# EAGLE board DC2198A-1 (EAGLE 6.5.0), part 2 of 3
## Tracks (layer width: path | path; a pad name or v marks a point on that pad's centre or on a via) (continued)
GND  (via drill 0.25) (continued)
  pour Top (no thermals): 50.29,32 46.74,32 46.74,35.31 51.56,35.31 52.2,34.67 52.2,33.02 51.56,33.02 51.56,34.42 51.31,34.67 50.55,34.67 50.29,34.42
  pour Bottom (no thermals): 50.29,32 46.74,32 46.74,35.18 49.91,35.18 50.29,34.8
  pour Bottom (no thermals): 69.6,41.27 69.6,36.58 67.44,36.58 67.06,36.2 67.06,35.05 65.15,35.05 65.15,36.58 65.53,36.96 65.53,40.26 66.55,41.27
  pour Top (no thermals): 61.85,32 58.29,32 58.29,35.31 63.12,35.31 63.75,34.67 63.75,33.02 63.12,33.02 63.12,34.42 62.87,34.67 62.1,34.67 61.85,34.42
  pour Bottom (no thermals): 61.85,32 58.29,32 58.29,35.18 61.47,35.18 61.85,34.8
  pour Bottom (no thermals): 81.15,41.27 81.15,36.58 78.99,36.58 78.61,36.2 78.61,35.05 76.71,35.05 76.71,36.58 77.09,36.96 77.09,40.26 78.11,41.27
  pour Top (no thermals): 73.41,32 69.85,32 69.85,35.31 74.68,35.31 75.31,34.67 75.31,33.02 74.68,33.02 74.68,34.42 74.42,34.67 73.66,34.67 73.41,34.42
  pour Bottom (no thermals): 73.41,32 69.85,32 69.85,35.18 73.03,35.18 73.41,34.8
  pour Bottom (no thermals): 92.71,41.27 92.71,36.58 90.55,36.58 90.17,36.2 90.17,35.05 88.27,35.05 88.27,36.58 88.65,36.96 88.65,40.26 89.66,41.27
  pour Top (no thermals): 84.96,32 81.41,32 81.41,35.31 86.23,35.31 86.87,34.67 86.87,33.02 86.23,33.02 86.23,34.42 85.98,34.67 85.22,34.67 84.96,34.42
  pour Bottom (no thermals): 84.96,32 81.41,32 81.41,35.18 84.58,35.18 84.96,34.8
  pour Bottom (no thermals): 104.27,41.27 104.27,36.58 102.11,36.58 101.73,36.2 101.73,35.05 99.82,35.05 99.82,36.58 100.2,36.96 100.2,40.26 101.22,41.27
  pour Top (no thermals): 96.52,32 92.96,32 92.96,35.31 97.79,35.31 98.42,34.67 98.42,33.02 97.79,33.02 97.79,34.42 97.54,34.67 96.77,34.67 96.52,34.42
  pour Bottom (no thermals): 96.52,32 92.96,32 92.96,35.18 96.14,35.18 96.52,34.8
  pour Top: 50.29,30.86 65.91,30.86 65.91,14.35 50.29,14.35
IBV_AUX  (via drill 0.25)
  Top 0.203: C20.1 110.4,24.42 110.57,24.59 112.47,24.59 113.03,25.15 113.03,26.04 112.14,26.92 112.14,27.34 U9.8 | 107.95,27.51 107.95,25.02 | U11.1 117.19,20.77 C25.1 | v113.41,21.21 113.41,21.03 114.17,20.77
  Top 0.254: U11.1 U11.2
  Top 0.406: C20.1 110.28,23.75 R28.2 108.71,22.23 108.08,22.23 108.08,22.99 C21.1 107.95,22.99 107.95,27.51 L9.2
  Top 1.016: 113.1,20.77 114.17,20.77 U11.1 | 108.71,22.23 108.71,21.59 109.78,20.77 113.1,20.77 | R30.2 113.2,20.73 113.16,20.83 113.1,20.77
  Bottom 0.406: D1.1 113.43,21.1 v113.41,21.21
  pour Top (no thermals): 107.06,19.81 107.06,26.42 106.68,26.8 105.66,26.8 105.66,28.32 107.82,28.32 108.33,27.81 108.33,24.51 111,24.51 111,21.46 119.38,21.46 119.38,19.94 119.25,19.81
INTVCC_LTC3604  (via drill 0.25)
  Top 0.203: v112.27,25.73 112.27,26.16 111.63,26.8 111.63,27.33 U9.7 | U9.1 108.99,29.94 108.97,29.97 v108.97,30.61 | U9.10 113.8,28.94 113.92,28.83 v113.92,25.4
  Bottom 0.203: C67.1 115.19,27.22 115.15,27.18 113.92,27.18 | 112.27,27.18 v112.27,25.73 | 112.27,27.18 109.09,27.18 108.97,27.3 v108.97,30.61 | 112.27,27.18 113.92,27.18 | 113.92,27.18 v113.92,25.4
ITH_LTC3604  (via drill 0.25)
  Top 0.203: U9.12 113.89,29.94 114.05,30.1 v114.05,30.86
  Bottom 0.203: v114.05,30.86 113.79,30.86 113.79,28.83 112.78,28.83 | 112.74,28.83 R102.2 112.78,28.83 | C68.1 110.49,28.57 112.78,28.57 112.78,28.83
N$1
  Top 0.406: P1.P 12.19,43.05 12.19,40.77 12.95,40.77 R17.1
N$2  (via drill 0.25)
  Top 0.203: v15.49,43.69 15.11,43.31 14.59,43.31 P1.N
  Bottom 0.203: v15.49,43.69 14.22,43.69 14.22,42.67 Q17.3
N$3
  Top 0.406: R26.2 LED1.P
N$4
  Top 0.406: P2.P 23.75,43.05 23.75,40.77 24.51,40.77 R18.1
N$5  (via drill 0.25)
  Top 0.203: v27.05,43.69 26.67,43.31 26.15,43.31 P2.N
  Bottom 0.203: v27.05,43.69 25.78,43.69 25.78,42.67 Q16.3
N$6
  Top 0.406: P3.P 35.31,43.05 35.31,40.77 36.07,40.77 R19.1
N$7  (via drill 0.25)
  Top 0.203: v38.61,43.69 38.23,43.31 37.71,43.31 P3.N
  Bottom 0.203: v38.61,43.69 37.34,43.69 37.34,42.67 Q15.3
N$8
  Top 0.406: P4.P 46.86,43.05 46.86,40.77 47.62,40.77 R20.1
N$9  (via drill 0.25)
  Top 0.203: v50.16,43.69 49.78,43.31 49.26,43.31 P4.N
  Bottom 0.203: v50.16,43.69 48.9,43.69 48.9,42.67 Q14.3
N$10
  Top 0.406: P5.P 58.42,43.05 58.42,40.77 59.18,40.77 R21.1
N$11  (via drill 0.25)
  Top 0.203: v61.72,43.69 61.34,43.31 60.82,43.31 P5.N
  Bottom 0.203: v61.72,43.69 60.45,43.69 60.45,42.67 Q13.3
N$12
  Top 0.406: P6.P 69.98,43.05 69.98,40.77 70.74,40.77 R22.1
N$13  (via drill 0.25)
  Top 0.203: v73.28,43.69 72.9,43.31 72.38,43.31 P6.N
  Bottom 0.203: v73.28,43.69 72.01,43.69 72.01,42.67 Q12.3
N$14
  Top 0.406: P7.P 81.53,43.05 81.53,40.77 82.3,40.77 R23.1
N$15  (via drill 0.25)
  Top 0.203: v84.84,43.69 84.45,43.31 83.94,43.31 P7.N
  Bottom 0.203: v84.84,43.69 83.57,43.69 83.57,42.67 Q11.3
N$16
  Top 0.406: P8.P 93.09,43.05 93.09,40.77 93.85,40.77 R24.1
N$17  (via drill 0.25)
  Top 0.203: v96.39,43.69 96.01,43.31 95.49,43.31 P8.N
  Bottom 0.203: v96.39,43.69 95.12,43.69 95.12,42.67 Q10.3
N$18  (via drill 0.25)
  Top 0.203: U21.16 113.67,11.01 113.67,11.05 114.55,11.05 v114.55,11.43 | R31.1 42.76,18.2 42.93,18.03 42.93,13.72 v42.8,13.72
  Route15 0.203: v114.55,11.43 114.55,11.3 105.57,11.3 104.25,12.62 104.25,13.88 104,14.12 104,16.88 103.62,17.25 103.25,17.25 102.88,17.62 84.88,17.62 84.5,17.25 81.62,17.25 81.25,17.62 67,17.62 66.25,16.88 64.88,16.88 64.5,16.5 64.5,16.12 63.62,15.25 63,15.25 62.62,14.88 62.62,13.62 62,13 55.12,13 54.75,13.38 46.62,13.38 46.38,13.12 43,13.12 42.8,13.32 42.8,13.33 42.8,13.34 v42.8,13.72
N$19
  Bottom 0.406: D1.3 113.03,20.45 112.27,21.21 C63.1 111.38,21.34 110.74,21.97 110.74,24.26 110.94,24.45 U23.4
N$20
  Bottom 0.203: R98.2 113.07,12.99 113.03,12.95 113.03,12.32 112.65,11.94 112.65,10.41 113.28,9.78 113.41,9.65 113.67,9.4 113.67,6.73 113.79,6.6 JP3.4
N$21  (via drill 0.25)
  Top 0.165: U10.K8 54.25,22.25 v54.25,23.25
  Bottom 0.165: v54.25,23.25 53.62,22.62 53.62,22.1 C90.2
N$22  (via drill 0.25)
  Top 0.165: U10.K2 v54.25,27.25
  Bottom 0.165: v54.25,27.25 52.88,27.25 52.88,26.69 C91.2
N$23  (via drill 0.25)
  Top 0.165: U10.J5 v56.25,25.25
  Bottom 0.165: v56.25,25.25 55.88,25.25 55.75,25.38 55.75,26.02 C92.1
N$24  (via drill 0.25)
  Top 0.165: U10.H5 v57.25,25.25
  Bottom 0.165: v57.25,25.25 57.25,26.15 C92.2
N$25  (via drill 0.25)
  Top 0.165: U10.J11 v56.25,19.25
  Bottom 0.165: v56.25,19.25 56.25,20.14 C93.1
N$26  (via drill 0.25)
  Top 0.165: U10.H2 U10.J2 v55.25,28.25
  Bottom 0.165: v55.25,28.25 55.25,29.15 C87.1
N$27  (via drill 0.25)
  Top 0.165: U10.H11 v57.25,19.25
  Bottom 0.165: C93.2 57.75,20.25 57.75,19.5 57.5,19.25 v57.25,19.25
N$29
  Top 0.406: P9.P 22.99,3.3 22.99,5.59 22.23,5.59 R39.1
N$30  (via drill 0.25)
  Top 0.203: v19.68,2.67 20.07,3.05 20.59,3.05 P9.N
  Bottom 0.203: v19.68,2.67 20.95,2.67 20.95,3.68 Q8.3
N$31
  Top 0.406: P10.P 34.54,3.3 34.54,5.59 33.78,5.59 R40.1
N$32  (via drill 0.25)
  Top 0.203: v31.24,2.67 31.62,3.05 32.14,3.05 P10.N
  Bottom 0.203: v31.24,2.67 32.51,2.67 32.51,3.68 Q7.3
N$33
  Top 0.406: P11.P 46.1,3.3 46.1,5.59 45.34,5.59 R41.1
N$34  (via drill 0.25)
  Top 0.203: v42.8,2.67 43.18,3.05 43.7,3.05 P11.N
  Bottom 0.203: v42.8,2.67 44.07,2.67 44.07,3.68 Q6.3
N$35
  Top 0.406: P12.P 57.66,3.3 57.66,5.59 56.9,5.59 R42.1
N$36  (via drill 0.25)
  Top 0.203: v54.36,2.67 54.74,3.05 55.26,3.05 P12.N
  Bottom 0.203: v54.36,2.67 55.63,2.67 55.63,3.68 Q5.3
N$37
  Top 0.406: P13.P 69.22,3.3 69.22,5.59 68.45,5.59 R43.1
N$38  (via drill 0.25)
  Top 0.203: v65.91,2.67 66.29,3.05 66.81,3.05 P13.N
  Bottom 0.203: v65.91,2.67 67.18,2.67 67.18,3.68 Q4.3
N$39
  Top 0.406: P14.P 80.77,3.3 80.77,5.59 80.01,5.59 R44.1
N$40  (via drill 0.25)
  Top 0.203: v77.47,2.67 77.85,3.05 78.37,3.05 P14.N
  Bottom 0.203: v77.47,2.67 78.74,2.67 78.74,3.68 Q3.3
N$41
  Top 0.406: P15.P 92.33,3.3 92.33,5.59 91.57,5.59 R45.1
N$42  (via drill 0.25)
  Top 0.203: v89.03,2.67 89.41,3.05 89.93,3.05 P15.N
  Bottom 0.203: v89.03,2.67 90.3,2.67 90.3,3.68 Q2.3
N$43
  Top 0.406: P16.P 103.63,3.3 103.89,3.56 103.89,5.59 103.12,5.59 R46.1
N$44  (via drill 0.25)
  Top 0.203: v100.58,2.67 100.97,3.05 101.48,3.05 P16.N
  Bottom 0.203: v100.58,2.67 101.85,2.67 101.85,3.68 Q1.3
N$57
  Top 0.406: R27.1 LED2.P
N$58  (via drill 0.25)
  Top 0.203: v14.78,26.67 15.74,26.67 LED1.N
  Bottom 0.203: U24.4 15.61,25.85 15.62,25.91 15.62,26.42 15.37,26.67 v14.78,26.67
N$60  (via drill 0.25)
  Top 0.203: v18.29,26.67 17.28,26.67 LED2.N
  Bottom 0.203: U24.6 16.98,25.61 16.89,25.78 16.89,26.42 17.13,26.66 18.28,26.66 v18.29,26.67
N$61
  Bottom 0.203: 112.78,31.46 C69.1
  Bottom 0.406: R102.1 112.78,31.46
N$63
  Top 0.254: LED3.P 106.55,19.43 106.55,18.25 R35.1
N$64  (via drill 0.25)
  Top 0.203: R34.2 121.92,18.33 121.92,18.92 121.41,19.43 v121.03,19.43 120.9,19.43 U11.5
  Route15 0.203: v121.03,19.43 116.46,19.43 115.95,18.92 113.92,18.92 113.67,19.18 113.67,19.94 114.05,20.32 115.19,20.32 116.33,21.46 v116.33,22.35
  Bottom 0.203: v116.33,22.35 R101.1
N$66
  Top 0.203: U21.4 109.81,8.29 109.22,7.7 109.22,7.24 108.71,6.73 108.71,5.08 108.97,4.83 112.42,4.83 112.62,4.65 113.08,4.65 114.28,5.84 115.82,5.84 116.33,5.33 118.53,5.33 C37.1 118.53,6.39 118.49,6.48 | 119.98,7.75 R38.2
  Top 0.254: 118.49,6.48 119,6.48 119,6.99 119.63,7.62 119.63,7.75 119.98,7.75
N$68
  Top 0.203: U11.4 120.4,19.56 120.4,18.29 120.4,18.33 R33.2
N$69
  Top 0.203: U11.6 121.4,20.08 121.79,19.68 122.43,19.68 122.81,19.3 122.81,17.4 122.68,17.27 119.63,17.27 119.51,17.4 119.51,19.18 | 119.89,20.76 U11.3 119.9,19.44 119.63,19.18 119.51,19.18 | 119.51,19.18 115.32,19.18 115.06,18.92 115.06,18.41 114.68,18.41 114.68,18.33 R32.2 | R30.1 113.16,18.29 R32.2 | R32.2 114.72,18.29
N$70
  Top 0.203: 110.89,25.63 110.89,25.59 C18.2 110.87,25.49 110.87,25.65 | 110.87,25.65 111,25.65 | 110.87,25.65 110.87,26.7 111.17,27 U9.6
N$74  (via drill 0.25)
  Top 0.203: R56.2 109.6,5.84 109.6,5.46 112.78,5.46 | 112.78,5.46 v112.78,5.33 | 112.78,5.46 113.03,5.46 113.16,5.59 U21.9 | U12.1 112.06,12.99 v112.27,13.21
  Bottom 0.203: v112.27,13.21 112.27,10.16 113.28,9.14 113.28,5.46 113.16,5.33 v112.78,5.33
RESETB  (via drill 0.25)
  Top 0.165: TP22.TP 9.33,4.83 9.25,4.75 | 13.75,18.78 SW1.SW1 | U10.L9 53.25,21.25 v51.5,21.25 49,21.25 48.62,21.62 43.38,21.62 42.25,20.5 36.62,20.5 36.12,20 35.75,20 | v51,26.5 51,27 51.25,27.25 53.25,27.25 U10.L3 | 35.75,20 14.22,20 | v35.75,19.75 35.75,20
  Top 0.203: SW1.SW1 14.73,18.92 | SW1.SW1 13.84,18.97 | C22.1 14.22,20 14.22,19.26 SW1.SW1
  Top 0.254: 9.25,4.75 7.01,6.99 7.01,16.38 7.51,16.88 13,16.88 13.75,17.62 13.75,18.78
  Route2 0.165: v65.38,19 64.38,18 55.75,18 54.62,19.12 51.75,19.12 51.5,19.38 v51.5,21.25
  Route15 0.165: v108.08,18.03 107.75,18.38 107,19.12 84.38,19.12 84,18.75 82.12,18.75 81.75,19.12 65.5,19.12 v65.38,19
  Bottom 0.165: v51.5,21.25 51.5,21.88 51.75,22.12 51.75,23.62 51.62,23.75 51.62,25 51,25.62 v51,26.5 | R136.R1_2 36.1,20.65 35.75,20.62 v35.75,19.75
  Bottom 0.203: 107.57,18.03 107.57,17.14 108.08,16.64 111.51,16.64 112.39,17.53 114.05,17.53 114.05,15.75 113.92,15.62 112.65,15.62 112.52,15.49 112.52,14.99 112.39,14.86 111.51,14.86 111.38,14.73 111.38,12.83 111.89,12.32 111.89,5.08 112.25,4.71 112.27,4.69 JP2.7 | 107.57,18.03 107.57,21.21 107.82,21.46 107.82,31.88 109.09,31.88 111.38,34.16 111.38,37.34 112.27,38.23 JP1.7 | v108.08,18.03 107.57,18.03
RUN_CH0
  Top 0.165: U10.B1 62.75,30.62 61.88,31.5 61.5,31.88 57.12,31.88 56.75,31.5 16.62,31.5 16.5,31.62 16.5,32.25 VSNSN1.1
  Top 0.203: U1.1 16.38,33.78 16.44,33.73 16.44,32.33 VSNSN1.1
  Bottom 0.203: R126.1 12.48,38.77 11.81,38.1 11.81,35.94 12.19,35.56 15.62,35.56 16.51,34.67 VSNSN1.1
  Bottom 0.406: Q17.1 12.23,42.02 12.19,41.91 12.19,40.39 R126.1
RUN_CH1  (via drill 0.25)
  Top 0.165: U10.C1 61.75,30.5 61.12,31.12 60.75,31.5 57.38,31.5 57,31.12 28.12,31.12 v28.12,31
  Top 0.203: U2.1 27.94,33.78 28,33.73 28,32.33 VSNSN2.1
  Bottom 0.165: v28.12,31 28.12,32.2 VSNSN2.1
  Bottom 0.203: R125.1 24.04,38.77 23.37,38.1 23.37,35.94 23.75,35.56 27.18,35.56 28.07,34.67 VSNSN2.1
  Bottom 0.406: Q16.1 23.79,42.02 23.75,41.91 23.75,40.39 R125.1
RUN_CH2  (via drill 0.25)
  Top 0.165: U10.D1 60.75,30.88 60.5,31.12 57.5,31.12 57.12,30.75 39.62,30.75 v39.62,30.62
  Top 0.203: U3.1 39.5,33.78 39.55,33.73 39.55,32.33 VSNSN3.1
  Bottom 0.165: v39.62,30.62 VSNSN3.1
  Bottom 0.203: R124.1 35.6,38.77 34.92,38.1 34.92,35.94 35.31,35.56 38.73,35.56 39.62,34.67 VSNSN3.1
  Bottom 0.406: Q15.1 35.34,42.02 35.31,41.91 35.31,40.39 R124.1
RUN_CH3  (via drill 0.25)
  Top 0.165: U10.J1 55.75,29.12 55.5,29.38 54.38,29.38 54.25,29.5 54.25,30.12 54,30.38 51.12,30.38 v51.12,30.25
  Top 0.203: U4.1 51.05,33.78 51.11,33.73 51.11,32.33 VSNSN4.1
  Bottom 0.165: v51.12,30.25 51.12,32.2 VSNSN4.1
  Bottom 0.203: R123.1 47.16,38.77 46.48,38.1 46.48,35.94 46.86,35.56 50.29,35.56 51.18,34.67 VSNSN4.1
  Bottom 0.406: Q14.1 46.9,42.02 46.86,41.91 46.86,40.39 R123.1
RUN_CH4  (via drill 0.25)
  Top 0.165: U10.H1 56.75,29.88 57.12,30.25 57.75,30.25 v58.12,30.62
  Top 0.203: U5.1 62.61,33.78 62.67,33.73 62.67,32.33 VSNSN5.1
  Bottom 0.165: v58.12,30.62 58.12,31.5 58.5,31.88 62.35,31.88 VSNSN5.1
  Bottom 0.203: R122.1 58.71,38.77 58.04,38.1 58.04,35.94 58.42,35.56 61.85,35.56 62.74,34.67 VSNSN5.1
  Bottom 0.406: Q13.1 58.46,42.02 58.42,41.91 58.42,40.39 R122.1
RUN_CH5  (via drill 0.25)
  Top 0.165: U10.E1 v59.75,29.38
  Top 0.203: U6.1 74.17,33.78 74.22,33.73 74.22,32.33 VSNSN6.1
  Route15 0.165: v59.75,29.38 60.38,29.38 61.38,30.38 70.25,30.38 70.62,30.75 74.25,30.75 v74.25,30.5
  Bottom 0.165: v74.25,30.5 74.25,32.21 VSNSN6.1
  Bottom 0.203: R121.1 70.27,38.77 69.6,38.1 69.6,35.94 69.98,35.56 73.41,35.56 74.3,34.67 VSNSN6.1
  Bottom 0.406: Q12.1 70.02,42.02 69.98,41.91 69.98,40.39 R121.1
RUN_CH6  (via drill 0.25)
  Top 0.165: U10.M1 v52.75,29.88
  Top 0.203: U7.1 85.72,33.78 85.78,33.73 85.78,32.33 VSNSN7.1
  Route15 0.165: v52.75,29.88 59,29.88 59.25,29.62 59.25,29.12 59.5,28.88 61.38,28.88 62.5,30 70.38,30 70.75,30.38 73.5,30.38 73.88,30 74.5,30 75.25,30.75 85.88,30.75 v85.88,30.5
  Bottom 0.165: v85.88,30.5 85.88,32.23 VSNSN7.1
  Bottom 0.203: R120.1 81.83,38.77 81.15,38.1 81.15,35.94 81.53,35.56 84.96,35.56 85.85,34.67 VSNSN7.1
  Bottom 0.406: Q11.1 81.57,42.02 81.53,41.91 81.53,40.39 R120.1
RUN_CH7  (via drill 0.25)
  Top 0.165: U10.L1 v53.75,29.38
  Top 0.203: U8.1 97.28,33.78 97.34,33.73 97.34,32.33 VSNSN8.1
  Route15 0.165: v53.75,29.38 53.75,29.5 58.75,29.5 58.88,29.38 58.88,29 59.38,28.5 61.5,28.5 62.62,29.62 74.75,29.62 75.38,30.25 85.38,30.25 85.62,30 86.12,30 86.38,30.25 89,30.25 89.88,31.12 97.38,31.12 v97.38,30.88
  Bottom 0.165: v97.38,30.88 97.38,32.22 VSNSN8.1
  Bottom 0.203: R119.1 93.38,38.77 92.71,38.1 92.71,35.94 93.09,35.56 96.52,35.56 97.41,34.67 VSNSN8.1
  Bottom 0.406: Q10.1 93.13,42.02 93.09,41.91 93.09,40.39 R119.1
RUN_CH8  (via drill 0.25)
  Top 0.165: U10.B7 63.25,23.25 70,23.25 v70.5,23.75
  Top 0.203: U13.1 18.8,12.57 18.74,12.63 18.74,14.03 VSNSN9.1
  Route15 0.165: v70.5,23.75 70.5,24.25 70.12,24.62 63.25,24.62 62.38,23.75 60.38,23.75 59.75,24.38 59.75,25.62 59.5,25.88 54,25.88 53.75,25.62 53.75,23 53.5,22.75 51.25,22.75 50.5,22 48.88,22 48,21.12 v18.75,21.12
  Bottom 0.165: v18.75,21.12 18.75,14.18 VSNSN9.1
  Bottom 0.203: R81.1 22.69,7.58 23.37,8.26 23.37,10.41 22.99,10.79 19.56,10.79 18.67,11.68 VSNSN9.1
  Bottom 0.406: Q8.1 22.95,4.33 22.99,4.45 22.99,5.97 R81.1
RUN_CH9  (via drill 0.25)
  Top 0.165: U10.C7 v61.25,22.25 | v48.5,22.5 48.5,22.12 48.38,22 43.25,22 42.12,20.88 35.38,20.88 34.62,21.62 v31.38,21.62
  Top 0.203: U14.1 30.42,14.03 30.35,14.1 VSNSN10.1
  Route2 0.165: v61.25,22.25 61,22.25 60.5,21.75 60,21.75 59.5,21.25 58,21.25 56.5,22.75 51.25,22.75 50.62,22.12 50.12,22.12 49.75,22.5 v48.5,22.5
  Bottom 0.165: v31.38,21.62 31.38,15.25 30.25,14.12 30.38,14.25 VSNSN10.1
  Bottom 0.203: R80.1 34.25,7.58 34.92,8.26 34.92,10.41 34.54,10.79 31.11,10.79 30.23,11.68 VSNSN10.1
  Bottom 0.406: Q7.1 34.51,4.33 34.54,4.45 34.54,5.97 R80.1
RUN_CH10  (via drill 0.25)
  Top 0.165: U10.D7 v60.25,22.25 | v47.62,22.5 47.62,22.88 47.25,23.25 43.38,23.25 v43.25,23.38
  Top 0.203: U15.1 41.98,14.03 41.91,14.1 VSNSN11.1
  Route2 0.165: v60.25,22.25 60,22.25 59.38,21.62 58.12,21.62 56.62,23.12 55.12,23.12 54.5,23.75 51.88,23.75 51.38,23.25 50.25,23.25 49.88,22.88 49.12,22.88 49,23 47.75,23 47.62,22.88 v47.62,22.5
  Bottom 0.165: v43.25,23.38 43.25,21.5 41.88,20.12 41.88,14.19 VSNSN11.1
  Bottom 0.203: R79.1 45.81,7.58 46.48,8.26 46.48,10.41 46.1,10.79 42.67,10.79 42.16,11.3 42.16,13.72 VSNSN11.1
  Bottom 0.406: Q6.1 46.06,4.33 46.1,4.45 46.1,5.97 R79.1
RUN_CH11  (via drill 0.25)
  Top 0.165: U10.J7 v55.25,22.25
  Top 0.203: U16.1 53.54,14.03 53.47,14.1 VSNSN12.1
  Bottom 0.165: v55.25,22.25 54.75,21.75 54.75,19 55.88,17.88 55.88,16.5 55.5,16.12 54.75,16.12 53.62,16.12 53.38,15.88 53.38,14.13 VSNSN12.1
  Bottom 0.203: R78.1 57.37,7.58 58.04,8.26 58.04,10.41 57.66,10.79 54.23,10.79 53.34,11.68 VSNSN12.1
  Bottom 0.406: Q5.1 57.62,4.33 57.66,4.45 57.66,5.97 R78.1
RUN_CH12  (via drill 0.25)
  Top 0.165: U10.H7 57.25,22.25 v57.25,21.25
  Top 0.203: U17.1 65.09,14.03 65.02,14.1 VSNSN13.1
  Bottom 0.165: v57.25,21.25 57.38,21.12 59.5,21.12 59.75,20.88 59.75,18.5 60.12,18.12 64.38,18.12 64.62,17.88 64.62,14.88 64.88,14.62 64.88,14.12 VSNSN13.1
  Bottom 0.203: R77.1 68.92,7.58 69.6,8.26 69.6,10.41 69.22,10.79 65.79,10.79 64.9,11.68 VSNSN13.1
  Bottom 0.406: Q4.1 69.18,4.33 69.22,4.45 69.22,5.97 R77.1
RUN_CH13  (via drill 0.25)
  Top 0.165: U10.E7 v59.25,22.25 | v66.38,22.75 66.5,22.88 70.5,22.88 71.38,23.75 v71.62,23.75
  Top 0.203: U18.1 76.65,14.03 76.58,14.1 VSNSN14.1
  Route15 0.165: v66.38,22.75 66.38,22.38 66.25,22.25 62.25,22.25 61.75,22.75 U10.E7 v59.25,22.25
  Bottom 0.165: v71.62,23.75 72.12,23.25 72.12,22 72,21.88 72,15.25 72.25,15 73.62,15 74.5,14.12 76.43,14.12 VSNSN14.1
  Bottom 0.203: R76.1 80.48,7.58 81.15,8.26 81.15,10.41 80.77,10.79 77.34,10.79 76.45,11.68 VSNSN14.1
  Bottom 0.406: Q3.1 80.73,4.33 80.77,4.45 80.77,5.97 R76.1
RUN_CH14  (via drill 0.25)
  Top 0.165: U10.M7 v50.5,22.75
  Top 0.203: U19.1 88.21,14.03 88.14,14.1 VSNSN15.1
  Route15 0.165: v50.5,22.75 51.5,23.75 52.62,23.75 52.88,24 52.88,25.75 53.75,26.62 60.75,26.62 61.62,25.75 62.5,25.75 62.88,25.38 73.25,25.38 73.75,25.88 88.38,25.88 89.75,24.5 v89.75,22.25
  Bottom 0.165: v89.75,22.25 89.75,15.25 89.38,14.88 88.25,14.88 88,14.62 88,14.09 VSNSN15.1
  Bottom 0.203: R75.1 92.04,7.58 92.71,8.26 92.71,10.41 92.33,10.79 88.9,10.79 88.01,11.68 VSNSN15.1
  Bottom 0.406: Q2.1 92.29,4.33 92.33,4.45 92.33,5.97 R75.1
RUN_CH15  (via drill 0.25)
  Top 0.165: U10.L7 53.25,22.25 50.25,22.25 49.62,22.88 v49.62,23.38 | v64.62,24.12 69,24.12 69.38,24.5 71.75,24.5 72.12,24.12 72.12,22.38 72.38,22.12 72.38,21.12 72.62,20.88 81.62,20.88 82,21.25 84.12,21.25 84.5,20.88 93,20.88 93.75,21.62 v99.12,21.62
  Top 0.203: U20.1 99.77,14.03 99.69,14.1 VSNSN16.1
  Route2 0.165: v49.62,23.38 49.62,23.5 49.75,23.62 51.12,23.62 51.62,24.12 54.38,24.12 55,24.75 55.5,24.75 55.75,24.5 55.75,23.75 56,23.5 56.75,23.5 57.5,22.75 64,22.75 64.62,23.38 v64.62,24.12
  Bottom 0.165: v99.12,21.62 99.5,21.25 99.5,14.16 VSNSN16.1
  Bottom 0.203: R74.1 103.59,7.58 104.27,8.26 104.27,10.41 103.89,10.79 100.46,10.79 99.57,11.68 VSNSN16.1
  Bottom 0.406: Q1.1 103.85,4.33 103.89,4.45 103.89,5.97 R74.1
SCL  (via drill 0.25)
  Top 0.165: U10.M12 v51.5,17.75 | v52.25,23.25 52.25,23.75 | U10.M6 52.25,23.75 | 52.25,23.75 52,24 43.88,24 42.38,25.5 v37.25,25.5 37.12,25.5 | 9.25,34.14 TP13.TP
  Top 0.203: U12.2 110.42,13.64 110.11,13.34 109.22,13.34 108.58,13.97 108.58,15.37 108.46,15.49 105.01,15.49 104.5,16 104.5,17.75 104,18.25 v103.5,18.25
  Top 0.305: 37.12,25.5 35.88,25.5 35.62,25.75 20.25,25.75 19.25,26.75 19.25,28.62 18.5,29.38 10.88,29.38 9.25,31 9.25,34.14
  Route15 0.165: v51.5,17.75 51.5,18.62 51.62,18.75 54.5,18.75 54.88,18.38 61.88,18.38 62.62,17.62 66,17.62 66.75,18.38 81.5,18.38 81.88,18 84.25,18 84.62,18.38 103.5,18.38 v103.5,18.25
  Bottom 0.165: v51.5,17.75 51.5,20.5 52.12,21.12 52.12,23.25 v52.25,23.25 | R137.R3_1 37.23,25.6 v37.25,25.5
SCL_IN  (via drill 0.25)
  Top 0.203: U12.3 110.83,14.22 113.28,14.22 | J2.4 129.24,17.64 128.34,16.74 126.56,16.74 125.95,16.13 113.28,16.13 | 113.28,14.22 113.28,13.21 112.14,12.06 112.14,11.02 U21.19 | v111.89,15.62 111.89,15.88 112.14,16.13 113.28,16.13 | 113.28,16.13 113.28,14.22
  Bottom 0.203: 111,16.26 107.7,16.26 107.06,16.89 107.06,21.46 107.44,21.84 107.44,32.26 108.84,32.26 110.87,34.29 110.87,37.59 111.28,37.95 111.28,40.12 JP1.6 | 111,16.26 111,12.45 111.51,11.94 111.51,5.08 111.28,4.85 111.28,2.18 110.87,1.78 110.31,1.78 110.31,1.72 JP2.6 | 111,16.26 111.89,16.26 | 111.89,16.26 112.27,16.64 R99.2 | 111.89,16.26 v111.89,15.62
SDA  (via drill 0.25)
  Top 0.165: U10.M5 51,24.75 | 51,24.75 44.12,24.75 42.38,26.5 38.25,26.5 38,26.25 37.25,26.25 | v37.25,26.38 37.25,26.25 | 37.25,26.25 20.5,26.25 19.75,27 v19.75,29.62 | v51,24.88 51,24.75 | v58.62,14.62 58.62,14.88 51.25,14.88 50.88,15.25 50.88,18.75 | U10.M11 50.88,18.75 | v50.88,19.5 50.88,18.75
  Top 0.203: 106.17,13.59 105.78,13.59 | U12.7 106.12,13.64 106.17,13.59 | 106.17,13.59 107.19,13.59 v107.19,13.34
  Route15 0.165: v58.62,14.62 58.62,14.88 60,14.88 60.5,15.38 61.5,15.38 61.75,15.62 63.5,15.62 64.12,16.25 64.12,16.62 64.75,17.25 66.12,17.25 66.88,18 81.38,18 81.75,17.62 84.38,17.62 84.75,18 103,18 103.38,17.62 104.12,17.62 104.38,17.38 104.38,15.38 104.88,14.88 105.62,14.88 107.12,13.38 v107.19,13.34
  Bottom 0.165: v19.75,29.62 19.38,29.62 18.38,30.62 9.62,30.62 9.25,30.25 9.25,26.95 TP14.TP | v50.88,19.5 51,19.62 51,21.88 51.38,22.25 51.38,23.25 51,23.62 v51,24.88 | R137.R2_1 36.85,26.4 v37.25,26.38
SDA_IN  (via drill 0.25)
  Top 0.203: U21.20 111.65,12.05 111.38,12.32 109.6,12.32 108.2,13.72 108.2,14.22 108.08,14.35 v107.19,14.35 106.18,14.35 U12.6 | 112.27,16.64 125.7,16.64 126.08,17.02 126.08,20.45 126.46,20.83 129,20.83 129.27,20.56 J2.2 | v109.47,13.97 109.22,13.97 108.97,14.22 108.97,16.26 109.35,16.64 112.27,16.64 | 112.27,16.64 112.27,19.05 112.01,19.3 v112.01,19.68
  Bottom 0.203: JP2.4 109.27,2.72 109.27,6.81 110.36,8 110.36,11.05 109.47,11.94 v109.47,13.97 107.57,13.97 v107.19,14.35 106.3,15.24 106.3,19.94 105.41,20.83 105.41,33.27 105.66,33.53 105.66,36.32 107.06,37.72 109.09,37.72 109.27,37.9 109.27,40.08 108.25,41.1 108.25,41.13 JP1.4
  Bottom 0.254: v112.01,19.68 112.52,19.68 112.9,19.3 112.9,18.41 R100.2
SHARE_CLK  (via drill 0.25)
  Top 0.165: U10.K9 v55.25,20.25 | U10.K3 55.25,26.25 v55.25,24.25
  Route15 0.165: v55.25,20.25 55.75,20.75 70.62,20.75 70.75,20.62 71.38,20.62 71.75,21 85.5,21 85.75,20.75 93.88,20.75 94.25,21.12 94.75,21.12 95.25,20.62 96.75,20.62 97.25,21.12 106,21.12 v106.12,21
  Route15 0.203: 109.27,2.72 | 109.27,2.72 107.31,2.72 v107.31,2.54 | JP2.5 109.27,2.72
  Bottom 0.165: v55.25,20.25 55.25,20.5 55.75,21 55.75,22.5 55.25,23 v55.25,24.25 55.25,24 52.12,24 52,24.12 52,25.25 51.5,25.75 51.5,26.75 51.25,27 50.12,27 49.75,26.62 38.75,26.62 38.12,26 38.12,22.75 37.77,22.4 R136.R3_2 | v106.12,21 106.12,20.95 106.62,20.95 106.68,21
  Bottom 0.203: 110.36,35.43 110.36,37.59 110.24,37.72 110.24,39.12 110.25,39.13 JP1.5 | JP2.5 110.25,3.72 110.25,7 110.74,7.49 110.74,11.3 110.24,11.81 110.24,14.22 109.73,14.73 107.82,14.73 106.68,15.88 106.68,21 106.68,21.72 107.06,22.1 107.06,32.64 108.58,32.64 110.36,34.42 110.36,35.43 | TP11.TP 110.36,35.43 | JP3.5 106.88,5.13 107.26,4.75 107.26,2.54 v107.31,2.54
SW1
  pour Top (no thermals): 22.1,33.02 17.91,33.02 17.91,34.67 22.1,34.67
SW2
  pour Top (no thermals): 33.66,33.02 29.46,33.02 29.46,34.67 33.66,34.67
SW3
  pour Top (no thermals): 45.21,33.02 41.02,33.02 41.02,34.67 45.21,34.67
SW4
  pour Top (no thermals): 56.77,33.02 52.58,33.02 52.58,34.67 56.77,34.67
SW5
  pour Top (no thermals): 68.33,33.02 64.14,33.02 64.14,34.67 68.33,34.67
SW6
  pour Top (no thermals): 79.88,33.02 75.69,33.02 75.69,34.67 79.88,34.67
SW7
  pour Top (no thermals): 91.44,33.02 87.25,33.02 87.25,34.67 91.44,34.67
SW8
  pour Top (no thermals): 103,33.02 98.81,33.02 98.81,34.67 103,34.67
SW11
  pour Top (no thermals): 13.08,13.34 17.27,13.34 17.27,11.68 13.08,11.68
SW12
  pour Top (no thermals): 24.64,13.34 28.83,13.34 28.83,11.68 24.64,11.68
SW13
  pour Top (no thermals): 36.2,13.34 40.39,13.34 40.39,11.68 36.2,11.68
SW14
  pour Top (no thermals): 47.75,13.34 51.94,13.34 51.94,11.68 47.75,11.68
SW15
  pour Top (no thermals): 59.31,13.34 63.5,13.34 63.5,11.68 59.31,11.68
SW16
  pour Top (no thermals): 70.87,13.34 75.06,13.34 75.06,11.68 70.87,11.68
SW17
  pour Top (no thermals): 82.42,13.34 86.61,13.34 86.61,11.68 82.42,11.68
SW18
  pour Top (no thermals): 93.98,13.34 98.17,13.34 98.17,11.68 93.98,11.68
SW_LTC3604
  Top 0.203: 109.16,25.37 C18.1
  pour Top (no thermals): 105.54,28.83 107.95,28.83 108.84,27.94 108.84,24.89 110.36,24.89 110.36,28.96 109.35,28.96 109.35,32 105.54,32
UNUSED1
  Route15 0.203: JP1.9 114.27,38.39 114.55,38.1 120.78,38.1 121.41,38.73 129.51,38.73 130.05,38.2 130.05,21.21 129.67,20.83 129.54,20.83 126.49,20.83 125.98,20.32 125.98,10.29 123.95,8.26 123.95,6.99 123.57,6.6 114.94,6.6 114.3,5.97 114.3,3.75 JP2.9
UNUSED2  (via drill 0.25)
  Top 0.203: v115.27,5.16 115.27,2.71 JP2.10
  Route15 0.203: JP1.10 114.3,41.13 114.3,41.91 114.81,42.42 119.38,42.42 120.14,41.66 120.14,40.51 121.41,39.24 129.67,39.24 130.56,38.35 130.56,9.4 129.79,8.64 125.09,8.64 124.59,8.13 124.59,6.86 123.83,6.1 115.7,6.1 115.32,5.71 115.32,5.21 v115.27,5.16
VDD  (via drill 0.25)
  Top 0.165: U10.G8 57.75,22.25 | 57.75,22.25 U10.G7 | v58.25,22.25 57.75,22.25 | U10.G1 U10.G2 57.75,28.25 v58.25,28.25
  Top 0.203: v101.85,7.75 103,7.75 103,7.11 103.04,7.24 R46.2 | v90.3,7.75 91.44,7.75 91.44,7.11 91.48,7.24 R45.2 | v78.74,7.75 79.88,7.75 79.88,7.11 79.92,7.24 R44.2 | v67.18,7.75 68.33,7.75 68.33,7.11 68.36,7.24 R43.2 | v55.63,7.75 56.77,7.75 56.77,7.11 56.81,7.24 R42.2 | v44.07,7.75 45.21,7.75 45.21,7.11 45.25,7.24 R41.2 | v32.51,7.75 33.66,7.75 33.66,7.11 33.69,7.24 R40.2 | v20.95,7.75 22.1,7.75 22.1,7.11 22.14,7.24 R39.2 | U11.16 U11.15 119.4,26.44 119.51,26.54 121.79,26.54 121.92,26.42 121.92,25.22 U11.10 U11.9 | TP20.TP1 110.24,17.14 109.22,17.14 108.46,16.38 106.89,16.38 R35.2 | v14.22,38.61 13.08,38.61 13.08,39.24 13.04,39.12 R17.2 | v25.78,38.61 24.64,38.61 24.64,39.24 24.6,39.12 R18.2 | v37.34,38.61 36.2,38.61 36.2,39.24 36.16,39.12 R19.2 | v48.9,38.61 47.75,38.61 47.75,39.24 47.71,39.12 R20.2 | v60.45,38.61 59.31,38.61 59.31,39.24 59.27,39.12 R21.2 | v72.01,38.61 70.87,38.61 70.87,39.24 70.83,39.12 R22.2 | v83.57,38.61 82.42,38.61 82.42,39.24 82.38,39.12 R23.2 | v95.12,38.61 93.98,38.61 93.98,39.24 93.94,39.12 R24.2
  Top 0.254: SW2.SW2 v33.53,18.92
  Bottom 0.203: 101.85,5.97 R74.2 | R75.2 90.3,5.97 | 78.74,5.97 R76.2 | 67.18,5.97 R77.2 | R78.2 55.63,5.97 | 44.07,5.97 R79.2 | R80.2 32.51,5.97 | 20.95,5.97 R81.2 | 14.22,40.39 R126.2 | 25.78,40.39 R125.2 | 37.34,40.39 R124.2 | 48.9,40.39 R123.2 | 60.45,40.39 R122.2 | 72.01,40.39 R121.2 | 83.57,40.39 R120.2 | 95.12,40.39 R119.2
  Bottom 0.305: v58.25,28.25 58.75,28.25 59.12,27.88 59.12,26.12 59.62,26.12 59.62,26.15 C86.1 | C89.1 58.23,22.35 v58.25,22.25
  Bottom 0.406: v101.85,7.75 101.85,5.97 | 90.3,5.97 v90.3,7.75 | v78.74,7.75 78.74,5.97 | v67.18,7.75 67.18,5.97 | 55.63,5.97 v55.63,7.75 | v44.07,7.75 44.07,5.97 | 32.51,5.97 v32.51,7.75 | v20.95,7.75 20.95,5.97 | v14.22,38.61 14.22,40.39 | v25.78,38.61 25.78,40.39 | v37.34,38.61 37.34,40.39 | v48.9,38.61 48.9,40.39 | v60.45,38.61 60.45,40.39 | v72.01,38.61 72.01,40.39 | v83.57,38.61 83.57,40.39 | v95.12,38.61 95.12,40.39
  other vias: 102.74,4.45 91.19,4.45 79.63,4.45 68.07,4.45 56.52,4.45 44.96,4.45 33.4,4.45 21.84,4.45 124.33,26.8 123.32,26.8 124.33,25.53 123.32,25.53 124.33,24.26 13.34,41.91 24.89,41.91 36.45,41.91 48.01,41.91 59.56,41.91 71.12,41.91 82.68,41.91 94.23,41.91 14,28.25
  pour Top (no thermals): 97.54,10.67 98.17,10.67 98.17,9.14 98.42,8.89 99.19,8.89 99.44,9.14 99.44,10.67 104.01,10.67 104.01,6.86 102.49,6.86 102.23,6.6 102.23,5.21 102.49,4.95 103.25,4.95 103.25,4.06 101.22,4.06 101.22,6.99 100.08,8.13 98.3,8.13 97.54,8.89
  pour Top (no thermals): 85.98,10.67 86.61,10.67 86.61,9.14 86.87,8.89 87.63,8.89 87.88,9.14 87.88,10.67 92.46,10.67 92.46,6.86 90.93,6.86 90.68,6.6 90.68,5.21 90.93,4.95 91.69,4.95 91.69,4.06 89.66,4.06 89.66,6.99 88.52,8.13 86.74,8.13 85.98,8.89
  pour Top (no thermals): 74.42,10.67 75.06,10.67 75.06,9.14 75.31,8.89 76.07,8.89 76.33,9.14 76.33,10.67 80.9,10.67 80.9,6.86 79.38,6.86 79.12,6.6 79.12,5.21 79.38,4.95 80.14,4.95 80.14,4.06 78.11,4.06 78.11,6.99 76.96,8.13 75.18,8.13 74.42,8.89
  pour Top (no thermals): 62.87,10.67 63.5,10.67 63.5,9.14 63.75,8.89 64.52,8.89 64.77,9.14 64.77,10.67 69.34,10.67 69.34,6.86 67.82,6.86 67.56,6.6 67.56,5.21 67.82,4.95 68.58,4.95 68.58,4.06 66.55,4.06 66.55,6.99 65.41,8.13 63.63,8.13 62.87,8.89
  pour Top (no thermals): 51.31,10.67 51.94,10.67 51.94,9.14 52.2,8.89 52.96,8.89 53.21,9.14 53.21,10.67 57.78,10.67 57.78,6.86 56.26,6.86 56.01,6.6 56.01,5.21 56.26,4.95 57.02,4.95 57.02,4.06 54.99,4.06 54.99,6.99 53.85,8.13 52.07,8.13 51.31,8.89
  pour Top (no thermals): 39.75,10.67 40.39,10.67 40.39,9.14 40.64,8.89 41.4,8.89 41.66,9.14 41.66,10.67 46.23,10.67 46.23,6.86 44.7,6.86 44.45,6.6 44.45,5.21 44.7,4.95 45.47,4.95 45.47,4.06 43.43,4.06 43.43,6.99 42.29,8.13 40.51,8.13 39.75,8.89
  pour Top (no thermals): 28.19,10.67 28.83,10.67 28.83,9.14 29.08,8.89 29.84,8.89 30.1,9.14 30.1,10.67 34.67,10.67 34.67,6.86 33.15,6.86 32.89,6.6 32.89,5.21 33.15,4.95 33.91,4.95 33.91,4.06 31.88,4.06 31.88,6.99 30.73,8.13 28.96,8.13 28.19,8.89
  pour Top (no thermals): 16.64,10.67 17.27,10.67 17.27,9.14 17.53,8.89 18.29,8.89 18.54,9.14 18.54,10.67 23.11,10.67 23.11,6.86 21.59,6.86 21.34,6.6 21.34,5.21 21.59,4.95 22.35,4.95 22.35,4.06 20.32,4.06 20.32,6.99 19.18,8.13 17.4,8.13 16.64,8.89
  pour Route15 (no thermals): 0.89,45.59 0.89,2.29 2.41,0.76 2.79,0.76 130.65,0.76 130.65,45.59
  pour Top (no thermals): 118.75,27.18 126.62,27.18 126.62,23.88 124.08,23.88 123.32,24.64 121.92,24.64 121.92,26.16 119.38,26.16 119.38,24.64 118.75,24.64
  pour Top (no thermals): 18.54,35.69 17.91,35.69 17.91,37.21 17.65,37.47 16.89,37.47 16.64,37.21 16.64,35.69 12.19,35.69 12.19,39.5 13.59,39.5 13.84,39.75 13.84,41.15 13.59,41.4 12.83,41.4 12.83,42.29 14.86,42.29 14.86,39.37 16,38.23 17.78,38.23 18.54,37.47
  pour Top (no thermals): 30.1,35.69 29.46,35.69 29.46,37.21 29.21,37.47 28.45,37.47 28.19,37.21 28.19,35.69 23.62,35.69 23.62,39.5 25.15,39.5 25.4,39.75 25.4,41.15 25.15,41.4 24.38,41.4 24.38,42.29 26.42,42.29 26.42,39.37 27.56,38.23 29.34,38.23 30.1,37.47
  pour Top (no thermals): 41.66,35.69 41.02,35.69 41.02,37.21 40.77,37.47 40.01,37.47 39.75,37.21 39.75,35.69 35.18,35.69 35.18,39.5 36.7,39.5 36.96,39.75 36.96,41.15 36.7,41.4 35.94,41.4 35.94,42.29 37.97,42.29 37.97,39.37 39.12,38.23 40.89,38.23 41.66,37.47
  pour Top (no thermals): 53.21,35.69 52.58,35.69 52.58,37.21 52.32,37.47 51.56,37.47 51.31,37.21 51.31,35.69 46.74,35.69 46.74,39.5 48.26,39.5 48.51,39.75 48.51,41.15 48.26,41.4 47.5,41.4 47.5,42.29 49.53,42.29 49.53,39.37 50.67,38.23 52.45,38.23 53.21,37.47
  pour Top (no thermals): 64.77,35.69 64.14,35.69 64.14,37.21 63.88,37.47 63.12,37.47 62.87,37.21 62.87,35.69 58.29,35.69 58.29,39.5 59.82,39.5 60.07,39.75 60.07,41.15 59.82,41.4 59.05,41.4 59.05,42.29 61.09,42.29 61.09,39.37 62.23,38.23 64.01,38.23 64.77,37.47
  pour Top (no thermals): 76.33,35.69 75.69,35.69 75.69,37.21 75.44,37.47 74.68,37.47 74.42,37.21 74.42,35.69 69.85,35.69 69.85,39.5 71.37,39.5 71.63,39.75 71.63,41.15 71.37,41.4 70.61,41.4 70.61,42.29 72.64,42.29 72.64,39.37 73.79,38.23 75.56,38.23 76.33,37.47
  pour Top (no thermals): 87.88,35.69 87.25,35.69 87.25,37.21 87,37.47 86.23,37.47 85.98,37.21 85.98,35.69 81.41,35.69 81.41,39.5 82.93,39.5 83.19,39.75 83.19,41.15 82.93,41.4 82.17,41.4 82.17,42.29 84.2,42.29 84.2,39.37 85.34,38.23 87.12,38.23 87.88,37.47
  pour Top (no thermals): 99.44,35.69 98.81,35.69 98.81,37.21 98.55,37.47 97.79,37.47 97.54,37.21 97.54,35.69 92.96,35.69 92.96,39.5 94.49,39.5 94.74,39.75 94.74,41.15 94.49,41.4 93.73,41.4 93.73,42.29 95.76,42.29 95.76,39.37 96.9,38.23 98.68,38.23 99.44,37.47
VFB1  (via drill 0.25)
  Top 0.203: U1.5 17.27,35.56 17.65,35.18 22.61,35.18 | 22.61,40.09 22.61,40.13 | 22.61,35.18 22.61,40.09 | v22.99,34.42 22.99,35.18 22.61,35.18 | 22.61,40.09 R9.2
  Top 0.254: R9.2 22.57,40.39
  Top 0.406: 22.57,40.39 C1.2 22.61,41.91 22.61,43.05 R1.1
  Bottom 0.203: v22.99,34.42 22.99,34.92 22.61,35.31 21.97,35.31 21.97,35.69 R117.1
VFB2  (via drill 0.25)
  Top 0.203: U2.5 28.83,35.56 29.21,35.18 34.16,35.18 | 34.16,40.09 34.16,40.13 | 34.16,35.18 34.16,40.09 | v34.54,34.42 34.54,35.18 34.16,35.18 | 34.16,40.09 R10.2
  Top 0.254: R10.2 34.12,40.39
  Top 0.406: 34.12,40.39 C2.2 34.16,41.91 34.16,43.05 R2.1
  Bottom 0.203: v34.54,34.42 34.54,34.92 34.16,35.31 33.53,35.31 33.53,35.69 R115.1
VFB3  (via drill 0.25)
  Top 0.203: U3.5 40.39,35.56 40.77,35.18 45.72,35.18 | 45.72,40.09 45.72,40.13 | 45.72,35.18 45.72,40.09 | v46.1,34.42 46.1,35.18 45.72,35.18 | 45.72,40.09 R11.2
  Top 0.254: R11.2 45.68,40.39
  Top 0.406: 45.68,40.39 C3.2 45.72,41.91 45.72,43.05 R3.1
  Bottom 0.203: v46.1,34.42 46.1,34.92 45.72,35.31 45.09,35.31 45.09,35.69 R113.1
VFB4  (via drill 0.25)
  Top 0.203: U13.5 17.91,10.79 17.53,11.18 12.57,11.18 | 12.57,6.26 12.57,6.22 | 12.57,6.26 12.57,11.18 | v12.19,11.94 12.19,11.18 12.57,11.18 | R48.2 12.57,6.26
  Top 0.254: 12.61,5.97 R48.2
  Top 0.406: 12.61,5.97 C38.2 12.57,4.45 12.57,3.3 R58.1
  Bottom 0.203: v12.19,11.94 12.19,11.43 12.57,11.05 13.21,11.05 13.21,10.67 R97.1
VFB5  (via drill 0.25)
  Top 0.203: U14.5 29.46,10.79 29.08,11.18 24.13,11.18 | 24.13,6.26 24.13,6.22 | 24.13,6.26 24.13,11.18 | v23.75,11.94 23.75,11.18 24.13,11.18 | R49.2 24.13,6.26
  Top 0.254: 24.17,5.97 R49.2
  Top 0.406: 24.17,5.97 C39.2 24.13,4.45 24.13,3.3 R59.1
  Bottom 0.203: v23.75,11.94 23.75,11.43 24.13,11.05 24.77,11.05 24.77,10.67 R95.1
VFB6  (via drill 0.25)
  Top 0.203: U15.5 41.02,10.79 40.64,11.18 35.69,11.18 | 35.69,6.26 35.69,6.22 | 35.69,6.26 35.69,11.18 | v35.31,11.94 35.31,11.18 35.69,11.18 | R50.2 35.69,6.26
  Top 0.254: 35.73,5.97 R50.2
  Top 0.406: 35.73,5.97 C40.2 35.69,4.45 35.69,3.3 R60.1
  Bottom 0.203: v35.31,11.94 35.31,11.43 35.69,11.05 36.32,11.05 36.32,10.67 R93.1
VFB7  (via drill 0.25)
  Top 0.203: U16.5 52.58,10.79 52.2,11.18 47.24,11.18 | 47.24,6.26 47.24,6.22 | 47.24,6.26 47.24,11.18 | v46.86,11.94 46.86,11.18 47.24,11.18 | R51.2 47.24,6.26
  Top 0.254: 47.28,5.97 R51.2
  Top 0.406: 47.28,5.97 C41.2 47.24,4.45 47.24,3.3 R61.1
  Bottom 0.203: v46.86,11.94 46.86,11.43 47.24,11.05 47.88,11.05 47.88,10.67 R91.1
VFB8  (via drill 0.25)
  Top 0.203: U17.5 64.14,10.79 63.75,11.18 58.8,11.18 | 58.8,6.26 58.8,6.22 | 58.8,6.26 58.8,11.18 | v58.42,11.94 58.42,11.18 58.8,11.18 | R52.2 58.8,6.26
  Top 0.254: 58.84,5.97 R52.2
  Top 0.406: 58.84,5.97 C42.2 58.8,4.45 58.8,3.3 R62.1
  Bottom 0.203: v58.42,11.94 58.42,11.43 58.8,11.05 59.44,11.05 59.44,10.67 R89.1
VFB9  (via drill 0.25)
  Top 0.203: U18.5 75.69,10.79 75.31,11.18 70.36,11.18 | 70.36,6.26 70.36,6.22 | 70.36,6.26 70.36,11.18 | v69.98,11.94 69.98,11.18 70.36,11.18 | R53.2 70.36,6.26
  Top 0.254: 70.4,5.97 R53.2
  Top 0.406: 70.4,5.97 C43.2 70.36,4.45 70.36,3.3 R63.1
  Bottom 0.203: v69.98,11.94 69.98,11.43 70.36,11.05 70.99,11.05 70.99,10.67 R87.1
VFB10  (via drill 0.25)
  Top 0.203: U19.5 87.25,10.79 86.87,11.18 81.92,11.18 | 81.92,6.26 81.92,6.22 | 81.92,6.26 81.92,11.18 | v81.53,11.94 81.53,11.18 81.92,11.18 | R54.2 81.92,6.26
  Top 0.254: 81.95,5.97 R54.2
  Top 0.406: 81.95,5.97 C44.2 81.92,4.45 81.92,3.3 R64.1
  Bottom 0.203: v81.53,11.94 81.53,11.43 81.92,11.05 82.55,11.05 82.55,10.67 R85.1
VFB11  (via drill 0.25)
  Top 0.203: U20.5 98.81,10.79 98.42,11.18 93.47,11.18 | 93.47,6.26 93.47,6.22 | 93.47,6.26 93.47,11.18 | v93.09,11.94 93.09,11.18 93.47,11.18 | R55.2 93.47,6.26
  Top 0.254: 93.51,5.97 R55.2
  Top 0.406: 93.51,5.97 C45.2 93.47,4.45 93.47,3.3 R65.1
  Bottom 0.203: v93.09,11.94 93.09,11.43 93.47,11.05 94.11,11.05 94.11,10.67 R83.1
VFB12  (via drill 0.25)
  Top 0.203: U4.5 51.94,35.56 52.32,35.18 57.28,35.18 | 57.28,40.09 57.28,40.13 | 57.28,35.18 57.28,40.09 | v57.66,34.42 57.66,35.18 57.28,35.18 | 57.28,40.09 R12.2
  Top 0.254: R12.2 57.24,40.39
  Top 0.406: 57.24,40.39 C4.2 57.28,41.91 57.28,43.05 R4.1
  Bottom 0.203: v57.66,34.42 57.66,34.92 57.28,35.31 56.64,35.31 56.64,35.69 R111.1
VFB13  (via drill 0.25)
  Top 0.203: U5.5 63.5,35.56 63.88,35.18 68.83,35.18 | 68.83,40.09 68.83,40.13 | 68.83,35.18 68.83,40.09 | v69.22,34.42 69.22,35.18 68.83,35.18 | 68.83,40.09 R13.2
  Top 0.254: R13.2 68.8,40.39
  Top 0.406: 68.8,40.39 C5.2 68.83,41.91 68.83,43.05 R5.1
  Bottom 0.203: v69.22,34.42 69.22,34.92 68.83,35.31 68.2,35.31 68.2,35.69 R109.1
VFB14  (via drill 0.25)
  Top 0.203: U6.5 75.06,35.56 75.44,35.18 80.39,35.18 | 80.39,40.09 80.39,40.13 | 80.39,35.18 80.39,40.09 | v80.77,34.42 80.77,35.18 80.39,35.18 | 80.39,40.09 R14.2
  Top 0.254: R14.2 80.35,40.39
  Top 0.406: 80.35,40.39 C6.2 80.39,41.91 80.39,43.05 R6.1
  Bottom 0.203: v80.77,34.42 80.77,34.92 80.39,35.31 79.76,35.31 79.76,35.69 R107.1
VFB15  (via drill 0.25)
  Top 0.203: U7.5 86.61,35.56 87,35.18 91.95,35.18 | 91.95,40.09 91.95,40.13 | 91.95,35.18 91.95,40.09 | v92.33,34.42 92.33,35.18 91.95,35.18 | 91.95,40.09 R15.2
  Top 0.254: R15.2 91.91,40.39
  Top 0.406: 91.91,40.39 C7.2 91.95,41.91 91.95,43.05 R7.1
  Bottom 0.203: v92.33,34.42 92.33,34.92 91.95,35.31 91.31,35.31 91.31,35.69 R105.1
VFB16  (via drill 0.25)
  Top 0.203: U8.5 98.17,35.56 98.55,35.18 103.5,35.18 | 103.5,40.09 103.5,40.13 | 103.5,35.18 103.5,40.09 | v103.76,34.8 103.76,35.18 103.5,35.18 | 103.5,40.09 R16.2
  Top 0.254: R16.2 103.47,40.39
  Top 0.406: 103.47,40.39 C8.2 103.5,41.91 103.5,43.05 R8.1
  Bottom 0.203: v103.76,34.8 103.76,35.05 103.5,35.31 102.87,35.31 102.87,35.69 R103.1
VOUT_CH0
  Top 0.254: R1.2 20.87,43.05 C1.1 17.4,41.91 TP3.TP
  pour Top (no thermals): 22.1,35.69 19.05,35.69 19.05,37.72 18.03,38.73 16.26,38.73 15.37,39.62 15.37,42.42 17.02,44.07 21.34,44.07 21.34,41.4 19.81,41.4 18.92,40.51 18.92,39.88 19.56,39.24 22.1,39.24
  pour Bottom (no thermals): 23.37,44.07 23.37,41.78 20.19,41.78 18.92,40.51 18.92,37.21 18.41,36.7 18.41,35.05 16.89,35.05 16,35.94 12.45,35.94 12.19,36.2 12.19,37.85 14.73,37.85 15.11,38.23 15.11,42.16 17.02,44.07
VOUT_CH1
  Top 0.254: R2.2 32.42,43.05 C2.1 28.96,41.91 TP4.TP
  pour Top (no thermals): 33.66,35.69 30.61,35.69 30.61,37.72 29.59,38.73 27.81,38.73 26.92,39.62 26.92,42.42 28.57,44.07 32.89,44.07 32.89,41.4 31.37,41.4 30.48,40.51 30.48,39.88 31.11,39.24 33.66,39.24
  pour Bottom (no thermals): 34.92,44.07 34.92,41.78 31.75,41.78 30.48,40.51 30.48,37.21 29.97,36.7 29.97,35.05 28.45,35.05 27.56,35.94 24,35.94 23.75,36.2 23.75,37.85 26.29,37.85 26.67,38.23 26.67,42.16 28.57,44.07
VOUT_CH2
  Top 0.254: R3.2 43.98,43.05 C3.1 40.51,41.91 TP5.TP
  pour Top (no thermals): 45.21,35.69 42.16,35.69 42.16,37.72 41.15,38.73 39.37,38.73 38.48,39.62 38.48,42.42 40.13,44.07 44.45,44.07 44.45,41.4 42.93,41.4 42.04,40.51 42.04,39.88 42.67,39.24 45.21,39.24
  pour Bottom (no thermals): 46.48,44.07 46.48,41.78 43.31,41.78 42.04,40.51 42.04,37.21 41.53,36.7 41.53,35.05 40.01,35.05 39.12,35.94 35.56,35.94 35.31,36.2 35.31,37.85 37.85,37.85 38.23,38.23 38.23,42.16 40.13,44.07
VOUT_CH3
  Top 0.254: R4.2 55.54,43.05 C4.1 52.07,41.91 TP6.TP
  pour Top (no thermals): 56.77,35.69 53.72,35.69 53.72,37.72 52.7,38.73 50.93,38.73 50.04,39.62 50.04,42.42 51.69,44.07 56.01,44.07 56.01,41.4 54.48,41.4 53.59,40.51 53.59,39.88 54.23,39.24 56.77,39.24
  pour Bottom (no thermals): 58.04,44.07 58.04,41.78 54.86,41.78 53.59,40.51 53.59,37.21 53.09,36.7 53.09,35.05 51.56,35.05 50.67,35.94 47.12,35.94 46.86,36.2 46.86,37.85 49.4,37.85 49.78,38.23 49.78,42.16 51.69,44.07
VOUT_CH4
  Top 0.254: R5.2 67.09,43.05 C5.1 63.63,41.91 TP7.TP
  pour Top (no thermals): 68.33,35.69 65.28,35.69 65.28,37.72 64.26,38.73 62.48,38.73 61.59,39.62 61.59,42.42 63.25,44.07 67.56,44.07 67.56,41.4 66.04,41.4 65.15,40.51 65.15,39.88 65.79,39.24 68.33,39.24
  pour Bottom (no thermals): 69.6,44.07 69.6,41.78 66.42,41.78 65.15,40.51 65.15,37.21 64.64,36.7 64.64,35.05 63.12,35.05 62.23,35.94 58.67,35.94 58.42,36.2 58.42,37.85 60.96,37.85 61.34,38.23 61.34,42.16 63.25,44.07
VOUT_CH5
  Top 0.254: R6.2 78.65,43.05 C6.1 75.18,41.91 TP8.TP
  pour Top (no thermals): 79.88,35.69 76.83,35.69 76.83,37.72 75.82,38.73 74.04,38.73 73.15,39.62 73.15,42.42 74.8,44.07 79.12,44.07 79.12,41.4 77.6,41.4 76.71,40.51 76.71,39.88 77.34,39.24 79.88,39.24
  pour Bottom (no thermals): 81.15,44.07 81.15,41.78 77.98,41.78 76.71,40.51 76.71,37.21 76.2,36.7 76.2,35.05 74.68,35.05 73.79,35.94 70.23,35.94 69.98,36.2 69.98,37.85 72.52,37.85 72.9,38.23 72.9,42.16 74.8,44.07
VOUT_CH6
  Top 0.254: R7.2 90.21,43.05 C7.1 86.74,41.91 TP9.TP
  pour Top (no thermals): 91.44,35.69 88.39,35.69 88.39,37.72 87.38,38.73 85.6,38.73 84.71,39.62 84.71,42.42 86.36,44.07 90.68,44.07 90.68,41.4 89.15,41.4 88.27,40.51 88.27,39.88 88.9,39.24 91.44,39.24
  pour Bottom (no thermals): 92.71,44.07 92.71,41.78 89.53,41.78 88.27,40.51 88.27,37.21 87.76,36.7 87.76,35.05 86.23,35.05 85.34,35.94 81.79,35.94 81.53,36.2 81.53,37.85 84.07,37.85 84.45,38.23 84.45,42.16 86.36,44.07
VOUT_CH7
  Top 0.254: R8.2 101.77,43.05 C8.1 98.3,41.91 TP10.TP
  pour Top (no thermals): 103,35.69 99.95,35.69 99.95,37.72 98.93,38.73 97.16,38.73 96.27,39.62 96.27,42.42 97.92,44.07 102.23,44.07 102.23,41.4 100.71,41.4 99.82,40.51 99.82,39.88 100.46,39.24 103,39.24
  pour Bottom (no thermals): 103.76,44.07 103.76,41.78 101.09,41.78 99.82,40.51 99.82,37.21 99.31,36.7 99.31,35.05 97.79,35.05 96.9,35.94 93.34,35.94 93.09,36.2 93.09,37.85 95.63,37.85 96.01,38.23 96.01,42.16 97.92,44.07
VOUT_CH8
  Top 0.254: R58.2 14.31,3.3 C38.1 17.78,4.45 TP23.TP
  pour Bottom (no thermals): 11.81,2.29 11.81,4.57 14.99,4.57 16.26,5.84 16.26,9.14 16.76,9.65 16.76,11.3 18.29,11.3 19.18,10.41 22.73,10.41 22.99,10.16 22.99,8.51 20.45,8.51 20.07,8.13 20.07,4.19 18.16,2.29
  pour Top (no thermals): 13.08,10.67 16.13,10.67 16.13,8.64 17.14,7.62 18.92,7.62 19.81,6.73 19.81,3.94 18.16,2.29 13.84,2.29 13.84,4.95 15.37,4.95 16.26,5.84 16.26,6.48 15.62,7.11 13.08,7.11
VOUT_CH9
  Top 0.254: R59.2 25.87,3.3 C39.1 29.34,4.45 TP24.TP
  pour Bottom (no thermals): 23.62,2.29 23.62,4.57 26.54,4.57 27.81,5.84 27.81,9.14 28.32,9.65 28.32,11.3 29.84,11.3 30.73,10.41 34.29,10.41 34.54,10.16 34.54,8.51 32,8.51 31.62,8.13 31.62,4.19 29.72,2.29
  pour Top (no thermals): 24.64,10.67 27.69,10.67 27.69,8.64 28.7,7.62 30.48,7.62 31.37,6.73 31.37,3.94 29.72,2.29 25.4,2.29 25.4,4.95 26.92,4.95 27.81,5.84 27.81,6.48 27.18,7.11 24.64,7.11
VOUT_CH10
  Top 0.254: R60.2 37.43,3.3 C40.1 40.89,4.45 TP25.TP
  Bottom 0.406: Q9.3 40.39,13.59 41.02,13.59 41.53,13.08 41.53,10.67 40.42,10.67 R92.1
  pour Bottom (no thermals): 35.18,2.29 35.18,4.57 38.1,4.57 39.37,5.84 39.37,9.14 39.88,9.65 39.88,11.3 41.4,11.3 42.29,10.41 45.85,10.41 46.1,10.16 46.1,8.51 43.56,8.51 43.18,8.13 43.18,4.19 41.27,2.29
  pour Top (no thermals): 36.2,10.67 39.24,10.67 39.24,8.64 40.26,7.62 42.04,7.62 42.93,6.73 42.93,3.94 41.27,2.29 36.96,2.29 36.96,4.95 38.48,4.95 39.37,5.84 39.37,6.48 38.73,7.11 36.2,7.11
VOUT_CH11
  Top 0.254: R61.2 48.98,3.3 C41.1 52.45,4.45 TP26.TP
  pour Bottom (no thermals): 46.74,2.29 46.74,4.57 49.66,4.57 50.93,5.84 50.93,9.14 51.44,9.65 51.44,11.3 52.96,11.3 53.85,10.41 57.4,10.41 57.66,10.16 57.66,8.51 55.12,8.51 54.74,8.13 54.74,4.19 52.83,2.29
  pour Top (no thermals): 47.75,10.67 50.8,10.67 50.8,8.64 51.82,7.62 53.59,7.62 54.48,6.73 54.48,3.94 52.83,2.29 48.51,2.29 48.51,4.95 50.04,4.95 50.93,5.84 50.93,6.48 50.29,7.11 47.75,7.11
VOUT_CH12
  Top 0.254: R62.2 60.54,3.3 C42.1 64.01,4.45 TP27.TP
  pour Bottom (no thermals): 58.29,2.29 58.29,4.57 61.21,4.57 62.48,5.84 62.48,9.14 62.99,9.65 62.99,11.3 64.52,11.3 65.41,10.41 68.96,10.41 69.22,10.16 69.22,8.51 66.67,8.51 66.29,8.13 66.29,4.19 64.39,2.29
  pour Top (no thermals): 59.31,10.67 62.36,10.67 62.36,8.64 63.37,7.62 65.15,7.62 66.04,6.73 66.04,3.94 64.39,2.29 60.07,2.29 60.07,4.95 61.59,4.95 62.48,5.84 62.48,6.48 61.85,7.11 59.31,7.11
VOUT_CH13
  Top 0.254: R63.2 72.1,3.3 C43.1 75.56,4.45 TP28.TP
  pour Top (no thermals): 70.87,10.67 73.91,10.67 73.91,8.64 74.93,7.62 76.71,7.62 77.6,6.73 77.6,3.94 75.95,2.29 71.63,2.29 71.63,4.95 73.15,4.95 74.04,5.84 74.04,6.48 73.41,7.11 70.87,7.11
  pour Bottom (no thermals): 69.85,2.29 69.85,4.57 72.77,4.57 74.04,5.84 74.04,9.14 74.55,9.65 74.55,11.3 76.07,11.3 76.96,10.41 80.52,10.41 80.77,10.16 80.77,8.51 78.23,8.51 77.85,8.13 77.85,4.19 75.95,2.29
VOUT_CH14
  Top 0.254: R64.2 83.65,3.3 C44.1 87.12,4.45 TP29.TP
  pour Bottom (no thermals): 81.41,2.29 81.41,4.57 84.33,4.57 85.6,5.84 85.6,9.14 86.11,9.65 86.11,11.3 87.63,11.3 88.52,10.41 92.08,10.41 92.33,10.16 92.33,8.51 89.79,8.51 89.41,8.13 89.41,4.19 87.5,2.29
  pour Top (no thermals): 82.42,10.67 85.47,10.67 85.47,8.64 86.49,7.62 88.27,7.62 89.15,6.73 89.15,3.94 87.5,2.29 83.19,2.29 83.19,4.95 84.71,4.95 85.6,5.84 85.6,6.48 84.96,7.11 82.42,7.11
VOUT_CH15
  Top 0.254: R65.2 95.21,3.3 C45.1 98.68,4.45 TP30.TP
  pour Bottom (no thermals): 92.96,2.29 92.96,4.57 95.89,4.57 97.16,5.84 97.16,9.14 97.66,9.65 97.66,11.3 99.19,11.3 100.08,10.41 103.63,10.41 103.89,10.16 103.89,8.51 101.35,8.51 100.97,8.13 100.97,4.19 99.06,2.29
  pour Top (no thermals): 93.98,10.67 97.03,10.67 97.03,8.64 98.04,7.62 99.82,7.62 100.71,6.73 100.71,3.94 99.06,2.29 94.74,2.29 94.74,4.95 96.27,4.95 97.16,5.84 97.16,6.48 96.52,7.11 93.98,7.11
VREF
  Bottom 0.406: U23.6 113.52,22.54 R101.2 113.67,22.35 113.67,24 C64.2
VSNSP_CH0  (via drill 0.25)
  Top 0.165: v19.5,31 19.5,30.75 19.75,30.5 27.38,30.5 27.75,30.12 28.62,30.12 28.88,30.38 38.38,30.38 39.12,29.62 40,29.62 40.38,30 49.12,30 49.38,29.75 49.38,29.38 49.38,28.25 v49.25,28.25 | v57.25,24.25 U10.G5
  Route2 0.165: v49.25,28.25 50,28.25 50.88,27.38 52.62,27.38 53.12,26.88 53.12,26.25 53.25,26.12 57.38,26.12 57.75,25.75 57.75,24.38 57.62,24.25 v57.25,24.25
  Bottom 0.165: VSNSN48.1 19.51,32.26 19.5,32.25 v19.5,31
  Bottom 0.203: 17.91,33.91 R118.2 | 19.56,33.91 C77.2
  Bottom 0.406: VSNSN48.1 19.56,33.91 17.91,33.91
VSNSP_CH1  (via drill 0.25)
  Top 0.165: U10.E5 v59.25,24.25
  Bottom 0.165: VSNSN46.1 31.11,31.76 31.5,31.38 38.62,31.38 38.75,31.25 38.75,30 39.12,29.62 40,29.62 40.5,30.12 40.5,30.62 40.75,30.88 49.62,30.88 49.75,30.75 49.75,28.5 50.88,27.38 51.62,27.38 51.88,27.12 51.88,26 52.12,25.75 54.62,25.75 55.62,24.75 57.88,24.75 58.38,24.25 v59.25,24.25
  Bottom 0.203: 29.46,33.91 R116.2 | 31.11,33.91 C76.2
  Bottom 0.406: VSNSN46.1 31.11,33.91 29.46,33.91
VSNSP_CH2  (via drill 0.25)
  Top 0.165: U10.A6 64.25,23.75 64.38,23.62 69.5,23.62 v69.5,23.75
  Route15 0.165: v69.62,31.62 69.62,31.5 42.88,31.5 42.75,31.62 42.75,32.18 VSNSN44.1
  Bottom 0.165: v69.5,23.75 69.62,23.75 v69.62,31.62
  Bottom 0.203: 41.02,33.91 R114.2 | 42.67,33.91 C75.2
  Bottom 0.406: VSNSN44.1 42.67,33.91 41.02,33.91
VSNSP_CH3  (via drill 0.25)
  Top 0.165: U10.B5 v62.25,25.25
  Bottom 0.165: v62.25,25.25 62.75,25.75 62.75,28 62.25,28.5 59.25,28.5 58.38,29.38 57.12,29.38 56,30.5 56,31.5 55.26,32.24 54.25,32.24 VSNSN42.1
  Bottom 0.203: 52.58,33.91 R112.2 | 54.23,33.91 C74.2
  Bottom 0.406: VSNSN42.1 54.23,33.91 52.58,33.91
VSNSP_CH4  (via drill 0.25)
  Top 0.165: U10.B4 63.25,26.25 v67,26.25
  Bottom 0.165: v67,26.25 67.12,26.25 67.5,26.62 67.5,31.5 66.78,32.22 65.75,32.22 VSNSN40.1
  Bottom 0.203: 64.14,33.91 R110.2 | 65.79,33.91 C73.2
  Bottom 0.406: VSNSN40.1 65.79,33.91 64.14,33.91
VSNSP_CH5  (via drill 0.25)
  Top 0.165: U10.C2 62.25,28.25 64.12,28.25 64.25,28.12 77.25,28.12 v77.38,28.25
  Bottom 0.165: v77.38,28.25 77.38,32.23 VSNSN38.1
  Bottom 0.203: 75.69,33.91 R108.2 | 77.34,33.91 C72.2
  Bottom 0.406: VSNSN38.1 77.34,33.91 75.69,33.91
VSNSP_CH6  (via drill 0.25)
  Top 0.165: U10.E2 59.25,28.25 v59.25,30.5
  Route15 0.165: v59.25,30.5 59.25,30.25 59.38,30.12 59.75,30.12 60,29.88 60.38,29.88 61.25,30.75 70.12,30.75 70.5,31.12 88.88,31.12 v88.88,30.88
  Bottom 0.165: v88.88,30.88 88.88,32.23 VSNSN36.1
  Bottom 0.406: R106.2 88.65,33.95 C71.2 88.9,33.95 VSNSN36.1
VSNSP_CH7  (via drill 0.25)
  Top 0.165: U10.A2 100,27.75 v100.38,28.12
  Bottom 0.165: v100.38,28.12 100.38,32.18 VSNSN34.1
  Bottom 0.203: 98.81,33.91 R104.2 | 100.46,33.91 C70.2
  Bottom 0.406: VSNSN34.1 100.46,33.91 98.81,33.91
VSNSP_CH8  (via drill 0.25)
  Top 0.165: U10.G11 v58.25,19.25
  Route15 0.165: v58.25,19.25 U10.G11 55,18.75 54.62,19.12 51.38,19.12 50.12,17.88 47.12,17.88 47,17.75 15.62,17.75 v15.62,18
  Bottom 0.165: v15.62,18 15.62,17.88 VSNSN31.1
  Bottom 0.203: 17.27,12.45 R96.2 | C62.2 15.62,12.45
  Bottom 0.406: VSNSN31.1 15.62,12.45 17.27,12.45
VSNSP_CH9  (via drill 0.25)
  Top 0.165: U10.E11 60.25,18.25 60.25,17.38 60.12,17.25 v60.12,16.5
  Route15 0.165: v60.12,16.5 59.5,16.5 59,16 48.75,16 48.38,16.38 47.75,16.38 47,15.62 27.12,15.62 v27.12,15.88
  Bottom 0.165: v27.12,15.88 27.12,14.15 VSNSN29.1
  Bottom 0.203: 28.83,12.45 R94.2 | C61.2 27.18,12.45
  Bottom 0.406: VSNSN29.1 27.18,12.45 28.83,12.45
VSNSP_CH10  (via drill 0.25)
  Top 0.165: U10.A12 v63.75,17
  Route15 0.165: v63.75,17 63.75,16.38 63.38,16 61.88,16 61.5,16.38 61.5,17.12 61.12,17.5 60,17.5 59,16.5 58.88,16.38 49,16.38 48.62,16.75 47.5,16.75 46.75,16 38.75,16 v38.75,16.25 38.75,16.38
  Bottom 0.165: VSNSN27.1 38.73,16.27 v38.75,16.25
  Bottom 0.203: 40.39,12.45 R92.2 | C60.2 38.73,12.45
  Bottom 0.406: VSNSN27.1 38.73,12.45 40.39,12.45
VSNSP_CH11  (via drill 0.25)
  Top 0.165: U10.B11 62.25,18.25 v62.25,16.5
  Route15 0.165: v62.25,16.5 62.25,17.5 61.88,17.88 56.12,17.88 55.75,17.5 55.75,17.25 55.62,17.12 49.5,17.12 v49.25,17.38
  Bottom 0.165: VSNSN25.1 50.25,14.1 50.25,14.12 49.5,14.12 49.25,14.38 v49.25,17.38
  Bottom 0.203: 51.94,12.45 R90.2 | C59.2 50.29,12.45
  Bottom 0.406: VSNSN25.1 50.29,12.45 51.94,12.45
VSNSP_CH12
